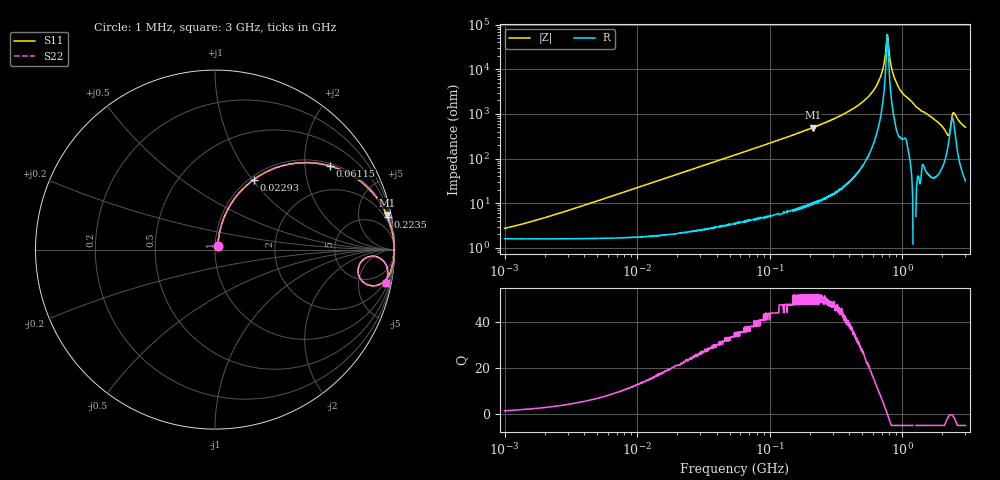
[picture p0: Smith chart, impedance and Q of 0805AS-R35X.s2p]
!s-Parameter Generated by FASTRON Sdn. Bhd.
!FASTRON P/N : 0805AS-R35X
!Keysight Technologies: E4991B_MY54100416_A.01.15
!Date: Mon Jun 15 12:54:38 2026
!Version  :Rev01  Mon Jun 15 12:54:38 2026
!Data & Calibration Information:
!Freq  S11  S21  S12  S22
!PortZ  Port1:50+j0  Port2:50+j0
!When reading reference impedance value at option line is always used.
! Remarks : This data is being provided solely for informational purposes.
# Hz S dB R 50
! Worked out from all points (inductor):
!   1601 points, 1 MHz to 3 GHz, reference 50 ohm
!   read as one part in series: L = 355 nH near 2.15 MHz
!   highest Q = 52.1 at 212.6 MHz (marker M1), where L = 371 nH
!   self-resonance near 773 MHz
!   S11 on the Smith chart (normalised r, x): 1 MHz: 1.03, +0.04; 22.93 MHz: 1.04, +1.02; 61.15 MHz: 1.08, +2.69; 223.5 MHz: 1, +11; 3 GHz: 2, -10
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1000000  -31.40 53.1  -0.14 -1.3  -0.14 -1.3  -31.40 53.1
3804036  -21.50 74.5  -0.17 -4.8  -0.17 -4.8  -21.50 74.5
1.447069e7  -10.40 69.2  -0.57 -17.5  -0.57 -17.5  -10.40 69.2
2.293104e7  -7.03 61.1  -1.15 -26.4  -1.15 -26.4  -7.03 61.1
5.504702e7  -2.38 38.9  -4.05 -49.5  -4.05 -49.5  -2.38 38.9
6.114642e7  -2.02 36.0  -4.60 -52.4  -4.60 -52.4  -2.02 36.0
2.083556e8  -0.21 11.6  -13.90 -77.3  -13.90 -77.3  -0.21 11.6
2.125681e8  -0.21 11.4  -14.10 -77.5  -14.10 -77.5  -0.21 11.4
2.234756e8  -0.19 10.7  -14.60 -78.1  -14.60 -78.1  -0.19 10.7
3.973271e8  -0.05 4.9  -21.30 -83.6  -21.30 -83.6  -0.05 4.9
5.611759e8  -0.02 2.3  -28.00 -85.0  -28.00 -85.0  -0.02 2.3
6.685918e8  -0.02 1.0  -34.90 -82.9  -34.90 -82.9  -0.02 1.0
7.135306e8  -0.02 0.6  -39.90 -79.0  -39.90 -79.0  -0.02 0.6
7.576891e8  -0.01 0.1  -50.30 -56.1  -50.30 -56.1  -0.01 0.1
7.925923e8  -0.01 -0.2  -48.90 62.1  -48.90 62.1  -0.01 -0.2
8.672962e8  -0.02 -0.8  -36.70 82.1  -36.70 82.1  -0.02 -0.8
1.02815e9  -0.04 -2.1  -28.70 82.0  -28.70 82.0  -0.04 -2.1
1.837163e9  -0.17 -8.4  -16.70 78.1  -16.70 78.1  -0.17 -8.4
2.167021e9  -1.03 -13.0  -12.40 56.1  -12.40 56.1  -1.03 -13.0
2.244273e9  -1.81 -10.0  -12.20 35.1  -12.20 35.1  -1.81 -10.0
2.455801e9  -0.48 -4.2  -20.90 51.3  -20.90 51.3  -0.48 -4.2
3e9  -0.27 -11.1  -14.30 75.3  -14.30 75.3  -0.27 -11.1
